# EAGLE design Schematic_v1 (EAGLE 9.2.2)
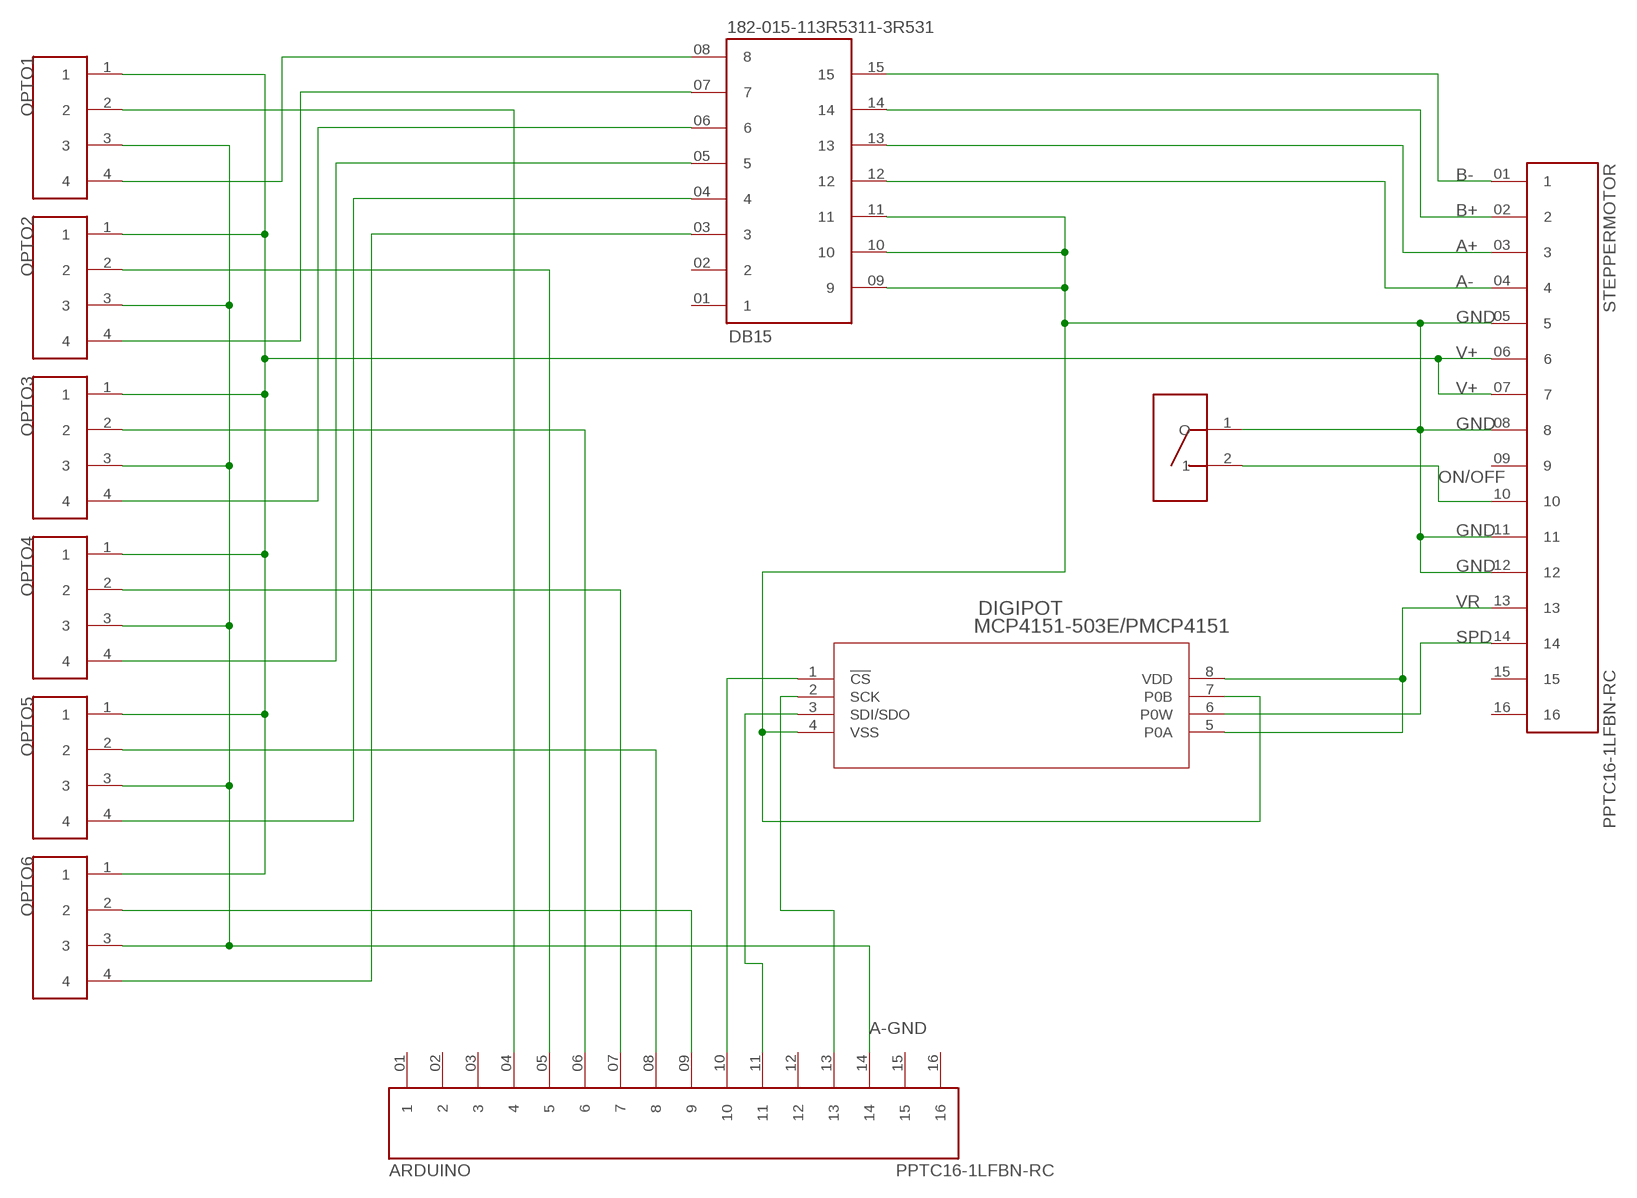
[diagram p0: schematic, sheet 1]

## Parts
ARDUINO  PPTC16-1LFBN-RC  [PPTC16-1]
DB15  182-015-113R5311-3R531  [182-015-1]
DIGIPOT  MCP4151-503E/PMCP4151  [PDIP8_300MC]
OPTO1  CPC1218IXYS  [CPC1218]
OPTO2  CPC1218IXYS  [CPC1218]
OPTO3  CPC1218IXYS  [CPC1218]
OPTO4  CPC1218IXYS  [CPC1218]
OPTO5  CPC1218IXYS  [CPC1218]
OPTO6  CPC1218IXYS  [CPC1218]
STEPPERMOTOR  PPTC16-1LFBN-RC  [PPTC16-1]
SWITCH  R1966ABLKBLKGR  [R1966]

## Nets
A+: DB15.13 STEPPERMOTOR.03
A-: DB15.12 STEPPERMOTOR.04
A-GND: ARDUINO.14 OPTO1.3 OPTO2.3 OPTO3.3 OPTO4.3 OPTO5.3 OPTO6.3
B+: DB15.14 STEPPERMOTOR.02
B-: DB15.15 STEPPERMOTOR.01
GND: DB15.09 DB15.10 DB15.11 DIGIPOT.4(VSS) DIGIPOT.7(P0B) STEPPERMOTOR.05 STEPPERMOTOR.08 STEPPERMOTOR.11 STEPPERMOTOR.12 SWITCH.1(O)
N$1: ARDUINO.13 DIGIPOT.2(SCK)
N$2: ARDUINO.11 DIGIPOT.3(SDI/SDO)
N$3: ARDUINO.10 DIGIPOT.1(!CS)
N$4: ARDUINO.04 OPTO1.2
N$5: ARDUINO.05 OPTO2.2
N$6: ARDUINO.06 OPTO3.2
N$7: ARDUINO.07 OPTO4.2
N$8: ARDUINO.08 OPTO5.2
N$9: ARDUINO.09 OPTO6.2
N$10: DB15.08 OPTO1.4
N$11: DB15.07 OPTO2.4
N$12: DB15.06 OPTO3.4
N$13: DB15.05 OPTO4.4
N$14: DB15.04 OPTO5.4
N$17: DB15.03 OPTO6.4
ON/OFF: STEPPERMOTOR.10 SWITCH.2
SPD: DIGIPOT.6(P0W) STEPPERMOTOR.14
V+: OPTO1.1 OPTO2.1 OPTO3.1 OPTO4.1 OPTO5.1 OPTO6.1 STEPPERMOTOR.06 STEPPERMOTOR.07
VR: DIGIPOT.5(P0A) DIGIPOT.8(VDD) STEPPERMOTOR.13
Unconnected: ARDUINO.01 ARDUINO.02 ARDUINO.03 ARDUINO.12 ARDUINO.15 ARDUINO.16 DB15.01 DB15.02 STEPPERMOTOR.09 STEPPERMOTOR.15 STEPPERMOTOR.16

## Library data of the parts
ARDUINO STEPPERMOTOR = HeaderPins:PPTC16-1
DB15 = DB15_Connector:182-015-113R531
DIGIPOT = MCP4151_DigiPotentiometer:MCP4151-503E/P; MANUFACTURER_PART_NUMBER: MCP4151503EP; VENDOR: Microchip
OPTO1-OPTO6 = Optoisolator:CPC1218
SWITCH = SPST_RockerSwitch:R1966

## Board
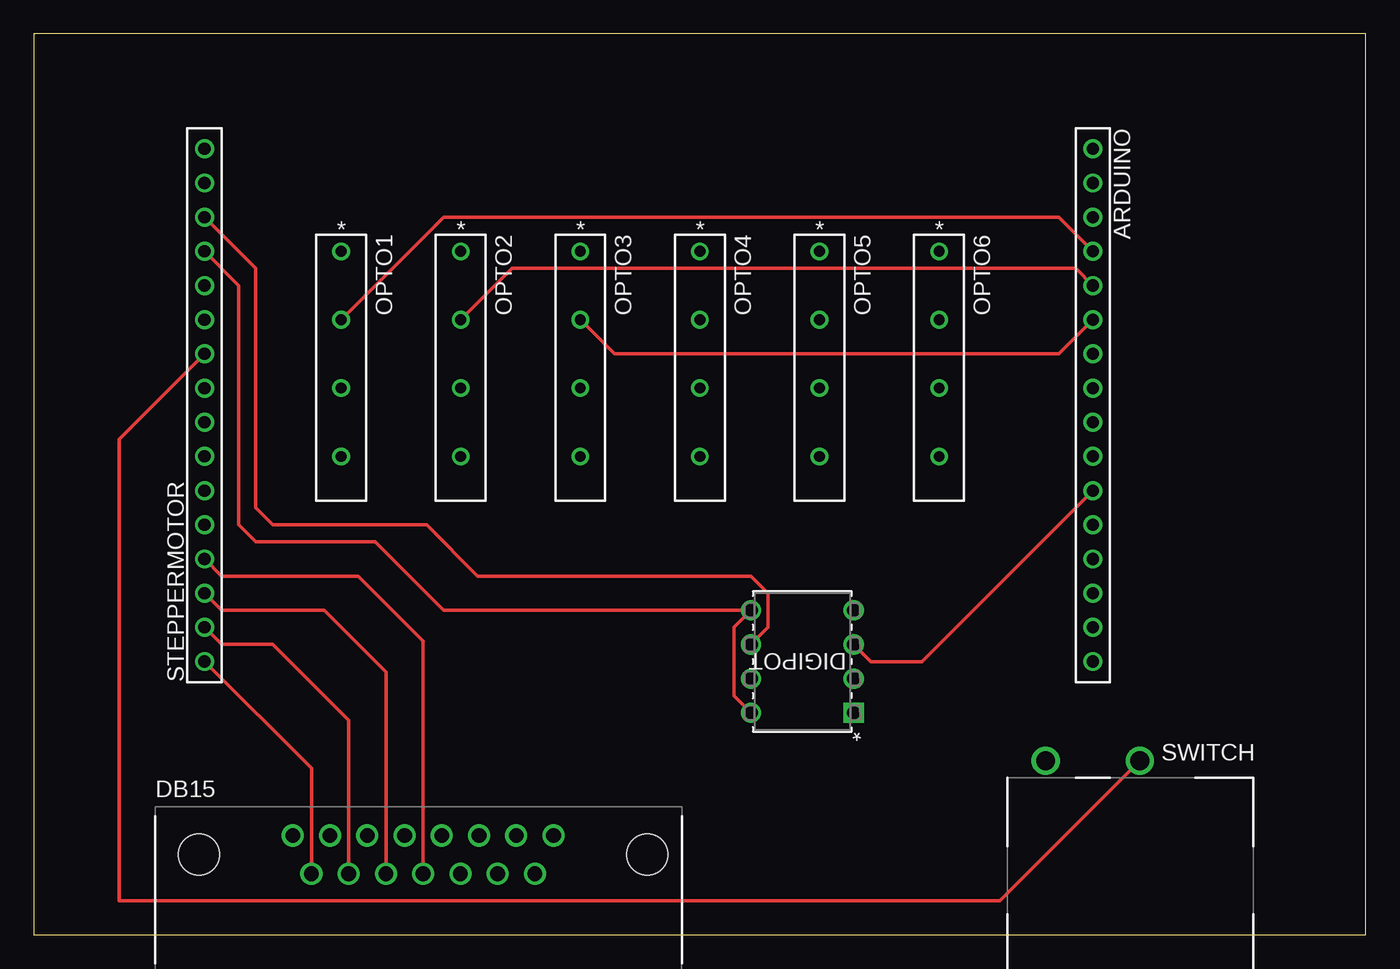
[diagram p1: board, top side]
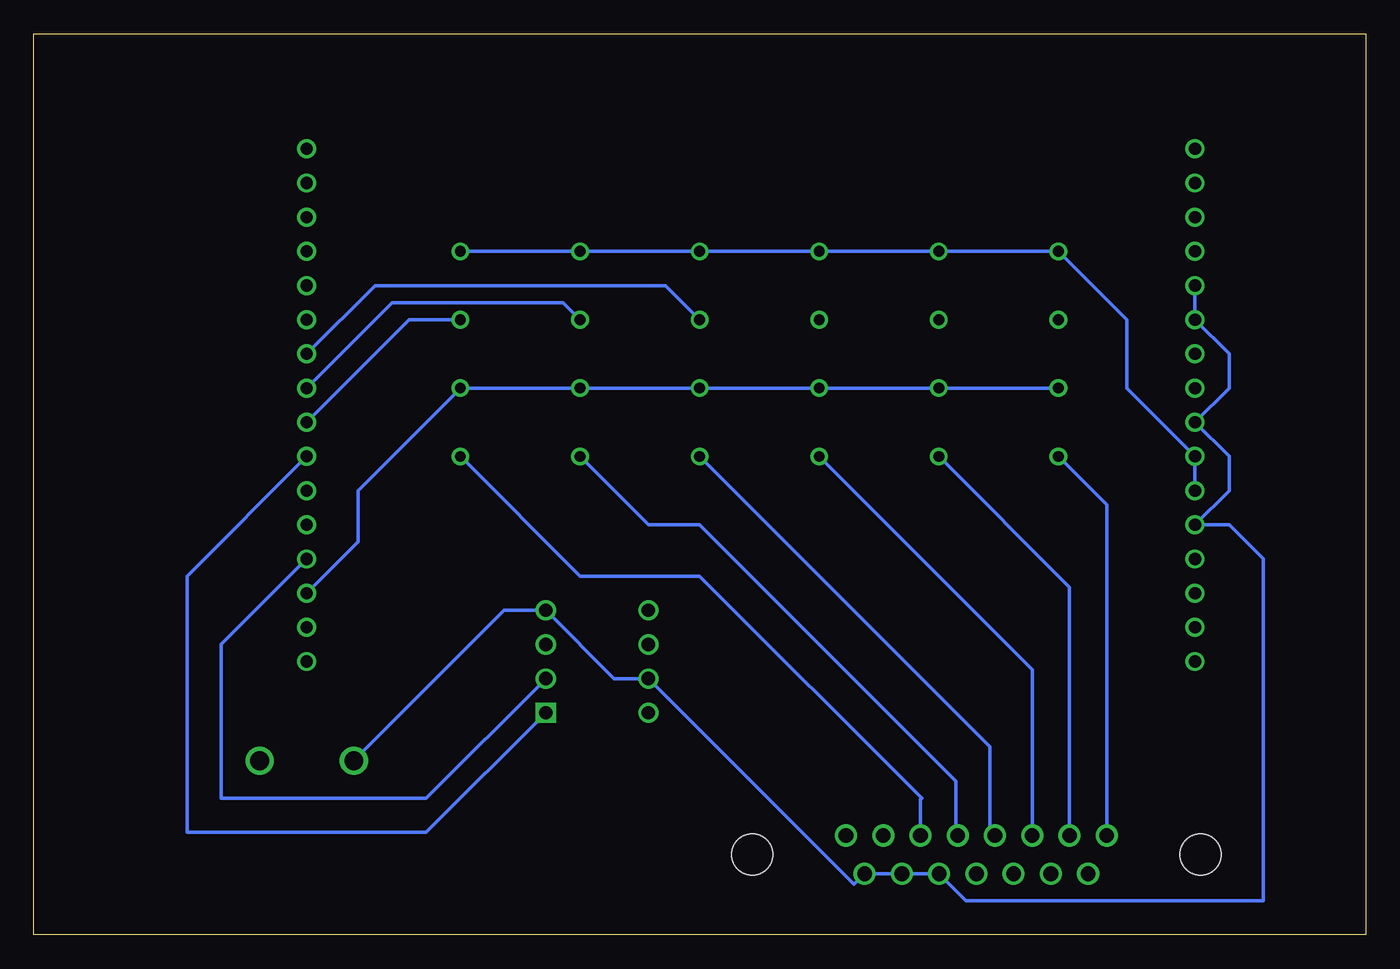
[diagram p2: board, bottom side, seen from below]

Size 99.04 x 66.98 mm. Coordinates in mm from the lower left corner, seen from the top.
Outline: 0,0 99.04,0 99.04,66.98 0,66.98 0,0
Copper layers (1*16): Top 0.035mm / dielectric 1.5mm / Bottom 0.035mm
Design rules "default": minimum track width 6mil, minimum drill 0.35mm, track to track 6mil, track to pad 6mil, pad to pad 6mil, via to via 6mil, smd to smd 6mil, copper to edge 40mil, drill to drill 6mil, minimum pad ring 10mil, minimum via ring 8mil, stop-mask expansion 4mil, vias tented up to drill 0mil, thermal gap 10mil

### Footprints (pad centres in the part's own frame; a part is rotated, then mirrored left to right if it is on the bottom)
PPTC16-1 = drill 0.9 pad 1.27: 01 -19.05,0; 02 -16.51,0; 03 -13.97,0; 04 -11.43,0; 05 -8.89,0; 06 -6.35,0; 07 -3.81,0; 08 -1.27,0; 09 1.27,0; 10 3.81,0; 11 6.35,0; 12 8.89,0; 13 11.43,0; 14 13.97,0; 15 16.51,0; 16 19.05,0
182-015-1 = drill 1.092 pad 1.524: 01 9.69,1.422; 02 6.921,1.422; 03 4.153,1.422; 04 1.384,1.422; 05 -1.384,1.422; 06 -4.153,1.422; 07 -6.921,1.422; 08 -9.69,1.422; 09 8.306,-1.422; 10 5.537,-1.422; 11 2.769,-1.422; 12 0,-1.422; 13 -2.769,-1.422; 14 -5.537,-1.422; 15 -8.306,-1.422 | hole 3.048: -16.662,0; 16.662,0
PDIP8_300MC = drill 0.991 pad 1.499 square: 1 -7.62,7.62 | drill 0.991 pad 1.499: 2 -7.62,5.08; 3 -7.62,2.54; 4 -7.62,0; 5 0,0; 6 0,2.54; 7 0,5.08; 8 0,7.62
CPC1218 = drill 0.8 pad 1.295: 1 -7.62,0; 2 -2.54,0; 3 2.54,0; 4 7.62,0
R1966 = drill 1.397: 1 -3.5,0; 2 3.5,0

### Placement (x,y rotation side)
ARDUINO  78.74,39.37 270 top
DB15  28.96,5.97 0 top
DIGIPOT  53.34,24.13 180 top
OPTO1  22.86,43.18 270 top
OPTO2  31.75,43.18 270 top
OPTO3  40.64,43.18 270 top
OPTO4  49.53,43.18 270 top
OPTO5  58.42,43.18 270 top
OPTO6  67.31,43.18 270 top
STEPPERMOTOR  12.7,39.37 90 top
SWITCH  78.74,12.95 0 top

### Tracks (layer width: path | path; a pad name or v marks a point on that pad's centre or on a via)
A+
  Top 0.254: STEPPERMOTOR.03 13.97,24.13 21.59,24.13 26.19,19.53 DB15.13
A-
  Top 0.254: DB15.12 28.96,21.84 24.13,26.67 13.97,26.67 STEPPERMOTOR.04
A-GND
  Bottom 0.254: OPTO1.3 OPTO2.3 OPTO3.3 OPTO4.3 OPTO5.3 OPTO6.3 74.93,33.02 74.93,29.21 ARDUINO.14
B+
  Top 0.254: STEPPERMOTOR.02 13.97,21.59 17.78,21.59 23.42,15.95 DB15.14
B-
  Top 0.254: STEPPERMOTOR.01 20.65,12.37 DB15.15
GND
  Bottom 0.254: STEPPERMOTOR.12 STEPPERMOTOR.11 10.16,43.18 10.16,40.64 STEPPERMOTOR.08 10.16,35.56 10.16,33.02 STEPPERMOTOR.05 10.16,30.48 7.62,27.94 7.62,2.54 29.72,2.54 DB15.11 DB15.10 DB15.09 38.05,3.76 DIGIPOT.7 55.88,19.05 DIGIPOT.4 64.06,24.13 SWITCH.1
N$1
  Bottom 0.254: DIGIPOT.2 69.85,10.16 85.09,10.16 85.09,21.59 ARDUINO.13
N$2
  Top 0.254: ARDUINO.11 66.04,20.32 62.23,20.32 DIGIPOT.3
N$3
  Bottom 0.254: DIGIPOT.1 69.85,7.62 87.63,7.62 87.63,26.67 ARDUINO.10
N$4
  Top 0.254: ARDUINO.04 76.2,53.34 30.48,53.34 OPTO1.2
N$5
  Top 0.254: ARDUINO.05 77.47,49.53 35.56,49.53 OPTO2.2
N$6
  Top 0.254: OPTO3.2 43.18,43.18 76.2,43.18 ARDUINO.06
N$7
  Bottom 0.254: OPTO4.2 52.07,48.26 73.66,48.26 ARDUINO.07
N$8
  Bottom 0.254: OPTO5.2 59.69,46.99 72.39,46.99 ARDUINO.08
N$9
  Bottom 0.254: OPTO6.2 71.12,45.72 ARDUINO.09
N$10
  Bottom 0.254: OPTO1.4 19.27,31.97 DB15.08
N$11
  Bottom 0.254: OPTO2.4 22.04,25.84 DB15.07
N$12
  Bottom 0.254: DB15.06 24.8,19.72 OPTO3.4
N$13
  Bottom 0.254: DB15.05 27.94,7.76 27.94,13.97 OPTO4.4
N$14
  Bottom 0.254: DB15.04 30.48,7.53 30.48,11.43 49.53,30.48 53.34,30.48 OPTO5.4
N$17
  Bottom 0.254: OPTO6.4 58.42,26.67 49.53,26.67 33.02,10.16 33.11,10.07 DB15.03
ON/OFF
  Top 0.254: STEPPERMOTOR.10 6.35,36.83 6.35,2.54 71.83,2.54 SWITCH.2
SPD
  Top 0.254: STEPPERMOTOR.14 16.51,49.53 16.51,31.75 17.78,30.48 29.21,30.48 33.02,26.67 53.34,26.67 54.61,25.4 54.61,22.86 DIGIPOT.6
V+
  Bottom 0.254: STEPPERMOTOR.06 STEPPERMOTOR.07 17.78,40.64 17.78,45.72 OPTO1.1 OPTO2.1 OPTO3.1 OPTO4.1 OPTO5.1 OPTO6.1
VR
  Top 0.254: STEPPERMOTOR.13 15.24,48.26 15.24,30.48 16.51,29.21 25.4,29.21 30.48,24.13 DIGIPOT.5 52.07,22.86 52.07,17.78 DIGIPOT.8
